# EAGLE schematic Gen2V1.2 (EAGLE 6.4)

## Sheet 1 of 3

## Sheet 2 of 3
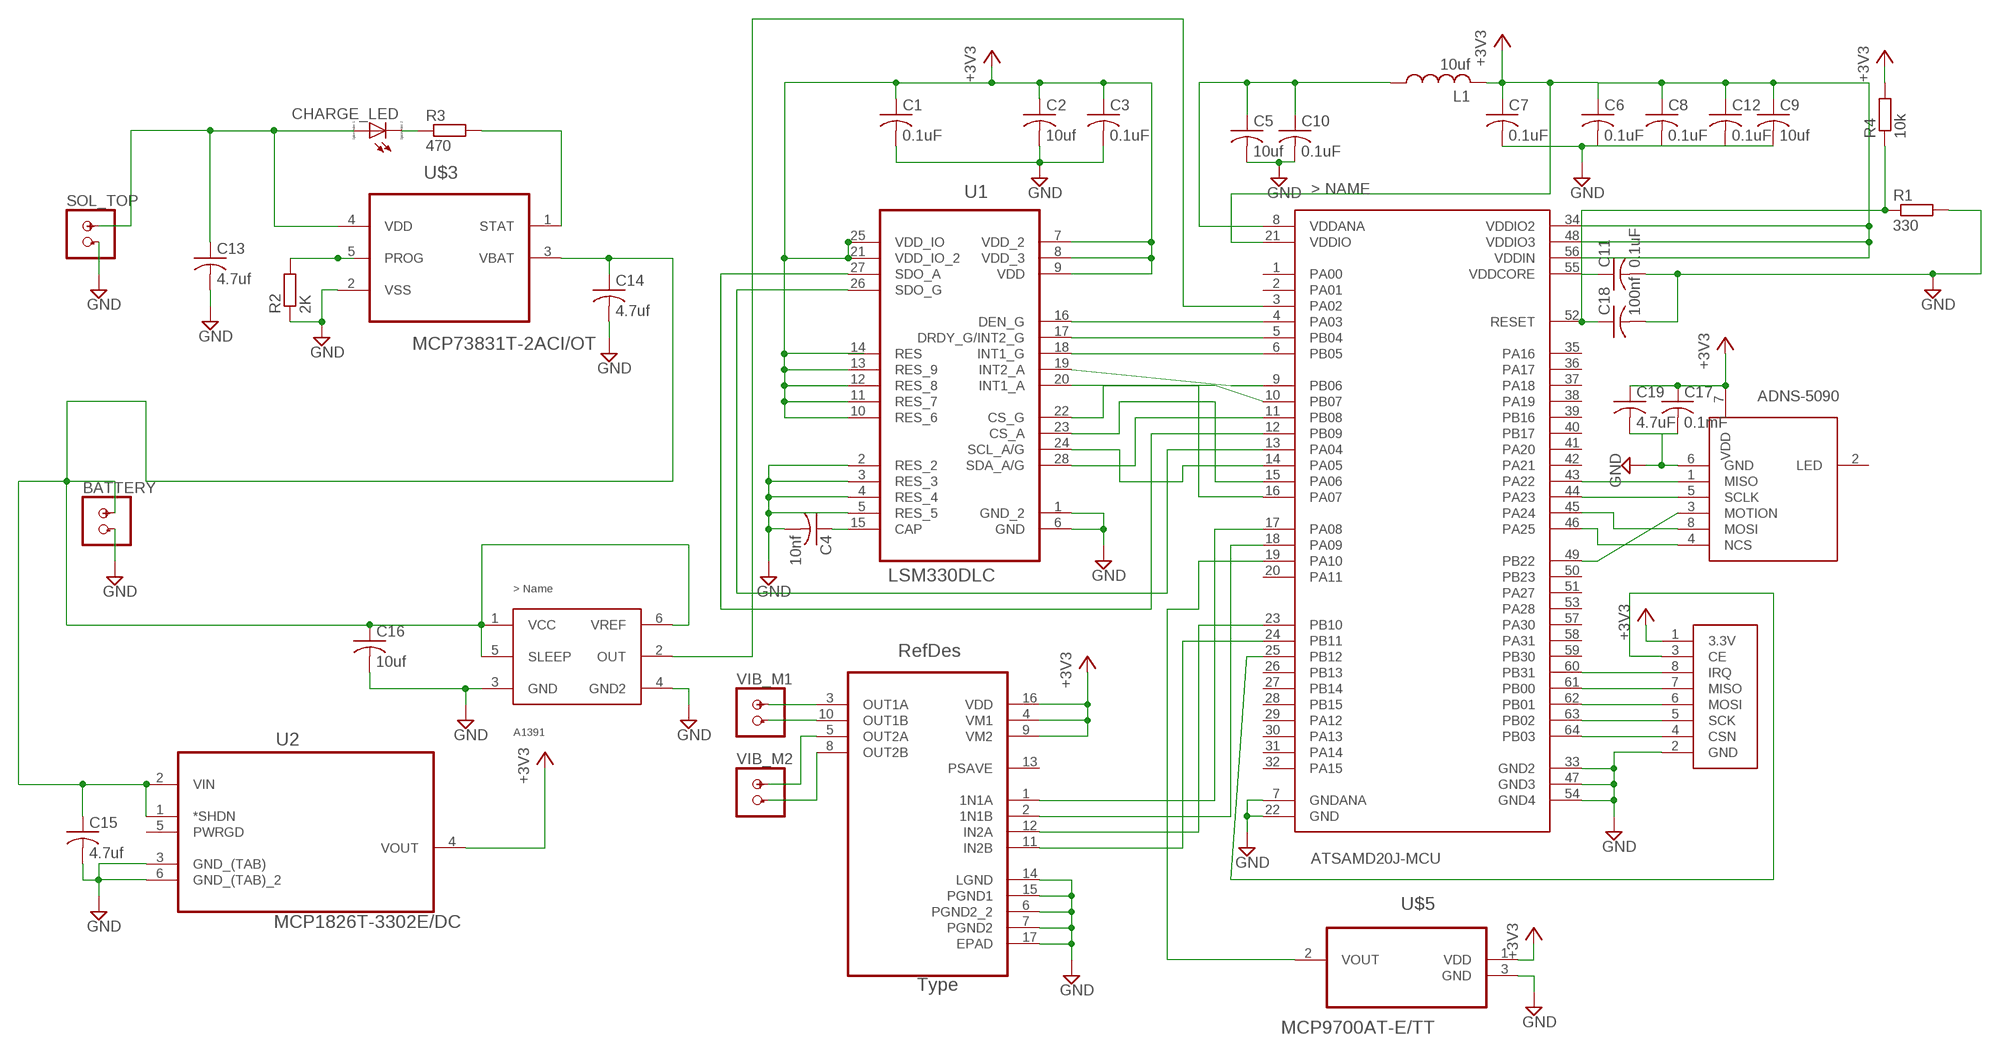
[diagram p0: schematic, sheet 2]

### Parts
BATTERY  PINHD-1X2POWER  [1X02]
C1  0.1uF  C-USC0402  [C0402]
C2  10uf  C-USC0402  [C0402]
C3  0.1uF  C-USC0402  [C0402]
C4  10nf  C-USC0402  [C0402]
C5  10uf  C-USC0402  [C0402]
C6  0.1uF  C-USC0402  [C0402]
C7  0.1uF  C-USC0402  [C0402]
C8  0.1uF  C-USC0402  [C0402]
C9  10uf  C-USC0402  [C0402]
C10  0.1uF  C-USC0402  [C0402]
C11  0.1uF  C-USC0402  [C0402]
C12  0.1uF  C-USC0402  [C0402]
C13  4.7uf  C-USC0402  [C0402]
C14  4.7uf  C-USC0402  [C0402]
C15  4.7uf  C-USC0402  [C0402]
C16  10uf  C-USC0402  [C0402]
C17  0.1mF  C-USC0402  [C0402]
C18  100nf  C-USC0402  [C0402]
C19  4.7uF  C-USC0402  [C0402]
CHARGE_LED  LED_E  [LED_1206]
L1  10uf  L-USWE-TPC  [POWER-CHOKE_WE-TPC]
R1  330  R-EU_R0805  [R0805]
R2  2K  R-EU_R0805  [R0805]
R3  470  R-EU_R0805  [R0805]
R4  10k  R-EU_R0805  [R0805]
SOL_TOP  PINHD-1X2POWER  [1X02]
U1  LSM330DLC  [LGA28R50P6X8_400X500X110]
U2  MCP1826T-3302E/DC  [SOT230P700X180-6N]
U3  MPC17C724EP  [QFN50P300X300X100-17N]
U$1  ATSAMD20J-MCU  [SAMD20JTQFP]
U$2  NRF24L01  [NRF24L01]
U$3  MCP73831T-2ACI/OT  [SOT95P280X145-5N]
U$4  A1391-CURRENTSENSOR  [A1391-CURRENTSENSOR]
U$5  MCP9700AT-E/TT  [SOT95P237X112-3N]
U$6  ADNS-5090  [ADNS-5090]
VIB_M1  PINHD-1X2MOTOR  [1X02/MOTOR]
VIB_M2  PINHD-1X2MOTOR  [1X02/MOTOR]

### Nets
+3V3: C1.1 C2.1 C3.1 C7.1 C17.1 C19.1 L1.2 R4.2 U1.7(VDD_2) U1.8(VDD_3) U1.9(VDD) U1.10(RES_6) U1.11(RES_7) U1.12(RES_8) U1.13(RES_9) U1.21(VDD_IO_2) U1.25(VDD_IO) U2.4(VOUT) U3.4(VM1) U3.9(VM2) U3.16(VDD) U$1.21(VDDIO) U$2.1(3.3V) U$5.1(VDD) U$6.7(VDD) ; also sheet 3
GND: BATTERY.2 C1.2 C2.2 C3.2 C4.2 C5.2 C6.2 C7.2 C8.2 C9.2 C10.2 C11.2 C12.2 C13.2 C14.2 C15.2 C16.2 C18.2 R1.2 R2.1 SOL_TOP.2 U1.1(GND_2) U1.2(RES_2) U1.3(RES_3) U1.4(RES_4) U1.5(RES_5) U1.6(GND) U2.3(GND_(TAB)) U2.6(GND_(TAB)_2) U3.6(PGND2_2) U3.7(PGND2) U3.14(LGND) U3.15(PGND1) U3.17(EPAD) U$1.7(GNDANA) U$1.22(GND) U$1.33(GND2) U$1.47(GND3) U$1.54(GND4) U$2.2(GND) U$3.2(VSS) U$4.3(GND) U$4.4(GND2) U$5.3(GND) U$6.6(GND) ; also sheet 3
N$1: U1.28(SDA_A/G) U$1.11(PB08)
N$2: U1.27(SDO_A) U$1.12(PB09)
N$3: U1.26(SDO_G) U$1.13(PA04)
N$4: U1.24(SCL_A/G) U$1.14(PA05)
N$5: U1.23(CS_A) U$1.15(PA06)
N$6: U1.22(CS_G) U$1.16(PA07)
N$7: U1.20(INT1_A) U$1.10(PB07)
N$8: U1.19(INT2_A) U$1.9(PB06)
N$9: C5.1 C10.1 L1.1 U$1.8(VDDANA)
N$10: C11.1 U$1.55(VDDCORE)
N$11: U$1.64(PB03) U$2.4(CSN)
N$12: U$1.63(PB02) U$2.5(SCK)
N$13: C6.1 C8.1 C9.1 C12.1 U$1.34(VDDIO2) U$1.48(VDDIO3) U$1.56(VDDIN)
N$14: U$1.61(PB00) U$2.7(MISO)
N$15: U$1.62(PB01) U$2.6(MOSI)
N$16: U$1.60(PB31) U$2.8(IRQ)
N$17: U$1.25(PB12) U$2.3(CE)
N$18: R2.2 U$3.5(PROG)
N$19: R3.2 U$3.1(STAT)
N$20: U3.2(1N1B) U$1.18(PA09)
N$21: CHARGE_LED.C R3.1
N$22: BATTERY.1 C14.1 C15.1 C16.1 U2.1(*SHDN) U2.2(VIN) U$3.3(VBAT) U$4.1(VCC) U$4.5(SLEEP) U$4.6(VREF)
N$23: U1.18(INT1_G) U$1.6(PB05)
N$24: U$1.3(PA02) U$4.2(OUT)
N$25: U3.1(1N1A) U$1.17(PA08)
N$26: U3.12(IN2A) U$1.23(PB10)
N$27: U3.11(IN2B) U$1.24(PB11)
N$28: U$1.19(PA10) U$5.2(VOUT)
N$29: U3.3(OUT1A) VIB_M1.1
N$30: U1.17(DRDY_G/INT2_G) U$1.5(PB04)
N$31: U1.16(DEN_G) U$1.4(PA03)
N$32: C4.1 U1.15(CAP)
N$33: U3.10(OUT1B) VIB_M1.2
N$34: C18.1 R1.1 R4.1 U$1.52(RESET)
N$35: U3.8(OUT2B) VIB_M2.2
N$36: C13.1 CHARGE_LED.A SOL_TOP.1 U$3.4(VDD)
N$37: U3.5(OUT2A) VIB_M2.1
N$38: U$1.46(PA25) U$6.4(NCS)
N$39: U$1.49(PB22) U$6.3(MOTION)
N$40: U$1.43(PA22) U$6.1(MISO)
N$41: U$1.44(PA23) U$6.5(SCLK)
N$42: U$1.45(PA24) U$6.8(MOSI)
N$43: C17.2 C19.2
Unconnected: U1.14(RES) U2.5(PWRGD) U3.13(PSAVE) U$1.1(PA00) U$1.2(PA01) U$1.20(PA11) U$1.26(PB13) U$1.27(PB14) U$1.28(PB15) U$1.29(PA12) U$1.30(PA13) U$1.31(PA14) U$1.32(PA15) U$1.35(PA16) U$1.36(PA17) U$1.37(PA18) U$1.38(PA19) U$1.39(PB16) U$1.40(PB17) U$1.41(PA20) U$1.42(PA21) U$1.50(PB23) U$1.51(PA27) U$1.53(PA28) U$1.57(PA30) U$1.58(PA31) U$1.59(PB30) U$6.2(LED)

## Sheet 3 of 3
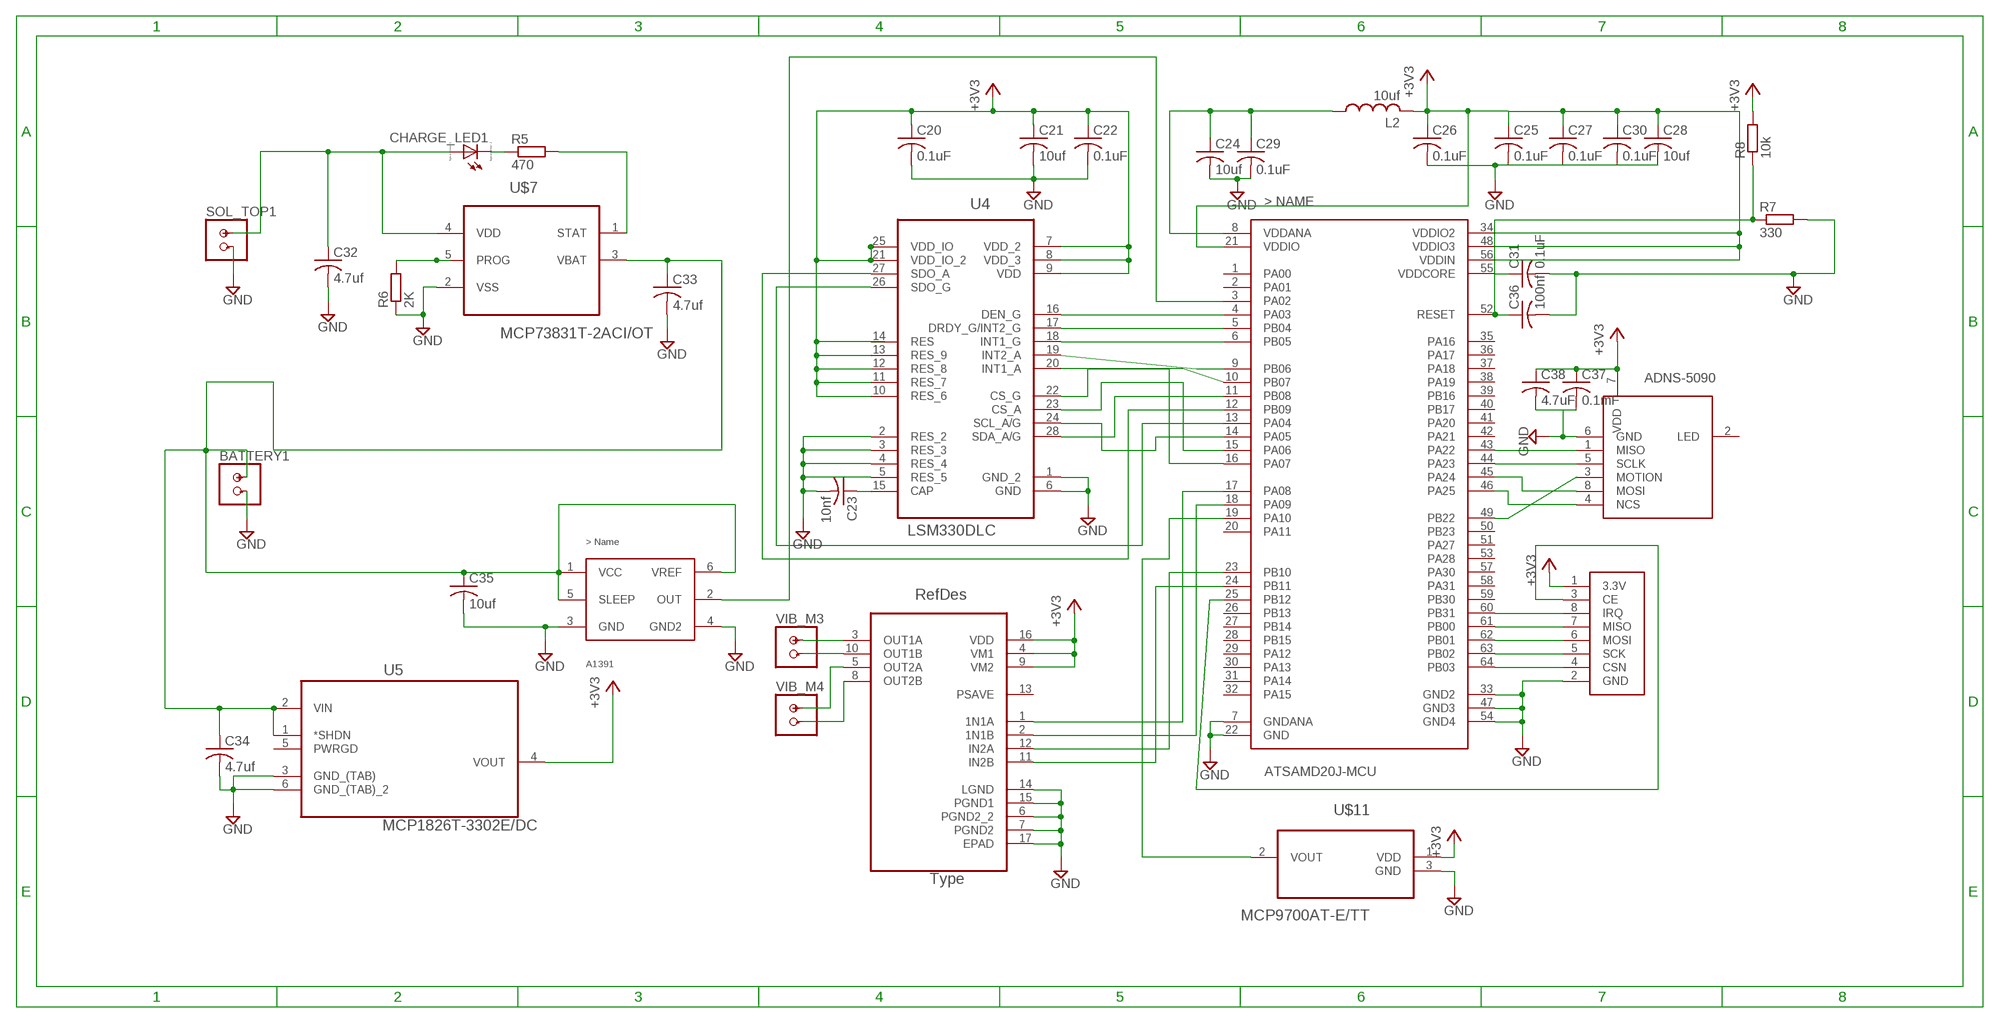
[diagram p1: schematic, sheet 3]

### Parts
BATTERY1  PINHD-1X2POWER  [1X02]
C20  0.1uF  C-USC0402  [C0402]
C21  10uf  C-USC0402  [C0402]
C22  0.1uF  C-USC0402  [C0402]
C23  10nf  C-USC0402  [C0402]
C24  10uf  C-USC0402  [C0402]
C25  0.1uF  C-USC0402  [C0402]
C26  0.1uF  C-USC0402  [C0402]
C27  0.1uF  C-USC0402  [C0402]
C28  10uf  C-USC0402  [C0402]
C29  0.1uF  C-USC0402  [C0402]
C30  0.1uF  C-USC0402  [C0402]
C31  0.1uF  C-USC0402  [C0402]
C32  4.7uf  C-USC0402  [C0402]
C33  4.7uf  C-USC0402  [C0402]
C34  4.7uf  C-USC0402  [C0402]
C35  10uf  C-USC0402  [C0402]
C36  100nf  C-USC0402  [C0402]
C37  0.1mF  C-USC0402  [C0402]
C38  4.7uF  C-USC0402  [C0402]
CHARGE_LED1  LED_E  [LED_1206]
L2  10uf  L-USWE-TPC  [POWER-CHOKE_WE-TPC]
R5  470  R-EU_R0805  [R0805]
R6  2K  R-EU_R0805  [R0805]
R7  330  R-EU_R0805  [R0805]
R8  10k  R-EU_R0805  [R0805]
SOL_TOP1  PINHD-1X2POWER  [1X02]
U4  LSM330DLC  [LGA28R50P6X8_400X500X110]
U5  MCP1826T-3302E/DC  [SOT230P700X180-6N]
U6  MPC17C724EP  [QFN50P300X300X100-17N]
U$7  MCP73831T-2ACI/OT  [SOT95P280X145-5N]
U$8  A1391-CURRENTSENSOR  [A1391-CURRENTSENSOR]
U$9  NRF24L01  [NRF24L01]
U$10  ATSAMD20J-MCU  [SAMD20JTQFP]
U$11  MCP9700AT-E/TT  [SOT95P237X112-3N]
U$12  ADNS-5090  [ADNS-5090]
VIB_M3  PINHD-1X2MOTOR  [1X02/MOTOR]
VIB_M4  PINHD-1X2MOTOR  [1X02/MOTOR]

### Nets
+3V3: C20.1 C21.1 C22.1 C26.1 C37.1 C38.1 L2.2 R8.2 U4.7(VDD_2) U4.8(VDD_3) U4.9(VDD) U4.10(RES_6) U4.11(RES_7) U4.12(RES_8) U4.13(RES_9) U4.21(VDD_IO_2) U4.25(VDD_IO) U5.4(VOUT) U6.4(VM1) U6.9(VM2) U6.16(VDD) U$9.1(3.3V) U$10.21(VDDIO) U$11.1(VDD) U$12.7(VDD) ; also sheet 2
GND: BATTERY1.2 C20.2 C21.2 C22.2 C23.2 C24.2 C25.2 C26.2 C27.2 C28.2 C29.2 C30.2 C31.2 C32.2 C33.2 C34.2 C35.2 C36.2 R6.1 R7.2 SOL_TOP1.2 U4.1(GND_2) U4.2(RES_2) U4.3(RES_3) U4.4(RES_4) U4.5(RES_5) U4.6(GND) U5.3(GND_(TAB)) U5.6(GND_(TAB)_2) U6.6(PGND2_2) U6.7(PGND2) U6.14(LGND) U6.15(PGND1) U6.17(EPAD) U$7.2(VSS) U$8.3(GND) U$8.4(GND2) U$9.2(GND) U$10.7(GNDANA) U$10.22(GND) U$10.33(GND2) U$10.47(GND3) U$10.54(GND4) U$11.3(GND) U$12.6(GND) ; also sheet 2
N$44: C24.1 C29.1 L2.1 U$10.8(VDDANA)
N$45: C31.1 U$10.55(VDDCORE)
N$46: C25.1 C27.1 C28.1 C30.1 U$10.34(VDDIO2) U$10.48(VDDIO3) U$10.56(VDDIN)
N$47: R6.2 U$7.5(PROG)
N$48: R5.2 U$7.1(STAT)
N$49: CHARGE_LED1.C R5.1
N$50: U$8.2(OUT) U$10.3(PA02)
N$51: C36.1 R7.1 R8.1 U$10.52(RESET)
N$52: C32.1 CHARGE_LED1.A SOL_TOP1.1 U$7.4(VDD)
N$53: BATTERY1.1 C33.1 C34.1 C35.1 U5.1(*SHDN) U5.2(VIN) U$7.3(VBAT) U$8.1(VCC) U$8.5(SLEEP) U$8.6(VREF)
N$54: U4.27(SDO_A) U$10.12(PB09)
N$55: U4.26(SDO_G) U$10.13(PA04)
N$56: U4.28(SDA_A/G) U$10.11(PB08)
N$57: U4.24(SCL_A/G) U$10.14(PA05)
N$58: U4.23(CS_A) U$10.15(PA06)
N$59: U4.22(CS_G) U$10.16(PA07)
N$60: U4.20(INT1_A) U$10.10(PB07)
N$61: U4.19(INT2_A) U$10.9(PB06)
N$62: U4.18(INT1_G) U$10.6(PB05)
N$63: U4.17(DRDY_G/INT2_G) U$10.5(PB04)
N$64: U4.16(DEN_G) U$10.4(PA03)
N$65: C23.1 U4.15(CAP)
N$66: U$9.4(CSN) U$10.64(PB03)
N$67: U$9.5(SCK) U$10.63(PB02)
N$68: U$9.8(IRQ) U$10.60(PB31)
N$69: U$9.7(MISO) U$10.61(PB00)
N$70: U$9.6(MOSI) U$10.62(PB01)
N$71: U$9.3(CE) U$10.25(PB12)
N$72: U6.2(1N1B) U$10.18(PA09)
N$73: U6.1(1N1A) U$10.17(PA08)
N$74: U6.12(IN2A) U$10.23(PB10)
N$75: U6.11(IN2B) U$10.24(PB11)
N$76: U$10.19(PA10) U$11.2(VOUT)
N$77: U6.3(OUT1A) VIB_M3.1
N$78: U6.10(OUT1B) VIB_M3.2
N$79: U6.8(OUT2B) VIB_M4.2
N$80: U6.5(OUT2A) VIB_M4.1
N$81: U$10.49(PB22) U$12.3(MOTION)
N$82: U$10.43(PA22) U$12.1(MISO)
N$83: U$10.44(PA23) U$12.5(SCLK)
N$84: U$10.45(PA24) U$12.8(MOSI)
N$85: U$10.46(PA25) U$12.4(NCS)
N$86: C37.2 C38.2
Unconnected: U4.14(RES) U5.5(PWRGD) U6.13(PSAVE) U$10.1(PA00) U$10.2(PA01) U$10.20(PA11) U$10.26(PB13) U$10.27(PB14) U$10.28(PB15) U$10.29(PA12) U$10.30(PA13) U$10.31(PA14) U$10.32(PA15) U$10.35(PA16) U$10.36(PA17) U$10.37(PA18) U$10.38(PA19) U$10.39(PB16) U$10.40(PB17) U$10.41(PA20) U$10.42(PA21) U$10.50(PB23) U$10.51(PA27) U$10.53(PA28) U$10.57(PA30) U$10.58(PA31) U$10.59(PB30) U$12.2(LED)

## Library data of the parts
BATTERY BATTERY1 SOL_TOP SOL_TOP1 VIB_M1-VIB_M4 = Custom 2 Pin Header:PINHD-1X2: PIN HEADER
C1-C38 = rcl:C-US: CAPACITOR, American symbol
CHARGE_LED CHARGE_LED1 = eagle-ltspice:LED_E: LED; SPICEMODEL: NONE; SPICEPREFIX: D; SPICETYPE: diode
L1 L2 = resistor:L-US: INDUCTOR, American symbol
R1-R8 = resistor:R-EU_: RESISTOR, European symbol
U1 U4 = LSM330DLC-IMU:LSM330DLC: ACC/GYRO, 3D, 16G, 2000DPS, 28LGA; MPN: LSM330DLC; OC_FARNELL: 2295820; OC_NEWARK: 68W6732; PACKAGE: LGA-28L; SUPPLIER: STMicroelectronics
U2 U5 = MCP1826T (3.3v Regulator):MCP1826T-3302E/DC: IC, LDO, 3.3V, 1A,; MPN: MCP1826T-3302E/DC; OC_FARNELL: 1578429; OC_NEWARK: 08N6499; PACKAGE: SOT223-5; SUPPLIER: Microchip
U3 U6 = MPC17C724EP-motordriver:MPC17C724EP: 0.4 A Dual H-Bridge Motor Driver IC; DESCRIPTION: 0.4 A Dual H-Bridge Motor Driver IC; MPN: MPC17C724EP; OC_FARNELL: -; OC_NEWARK: 53J3340; PACKAGE: QFN-16; SUPPLIER: FREESCALE SEMICONDUCTOR
U$1 U$10 = ATSAMD20J:ATSAMD20J-MCU
U$2 U$9 = SMD RF Module:NRF24L01: nrf24L01+
U$3 U$7 = MCP73831T (LiPo Charger):MCP73831T-2ACI/OT: Charge Management Controller; MPN: MCP73831T-2ACI/OT; OC_FARNELL: 1332158; OC_NEWARK: 56K7045; PACKAGE: SOT-5; SUPPLIER: Microchip
U$4 U$8 = A1391-halleffectcurrentsensor:A1391-CURRENTSENSOR
U$5 U$11 = MPC9700-tempsensor:MCP9700AT-E/TT: Low-Power Linear Active Thermistor; MPN: MCP9700AT-E/TT; OC_FARNELL: 1605577; OC_NEWARK: 84R5199; PACKAGE: SOT-3; SUPPLIER: MICROCHIP
U$6 U$12 = ADNS-5090(CMOS Camera):ADNS-5090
